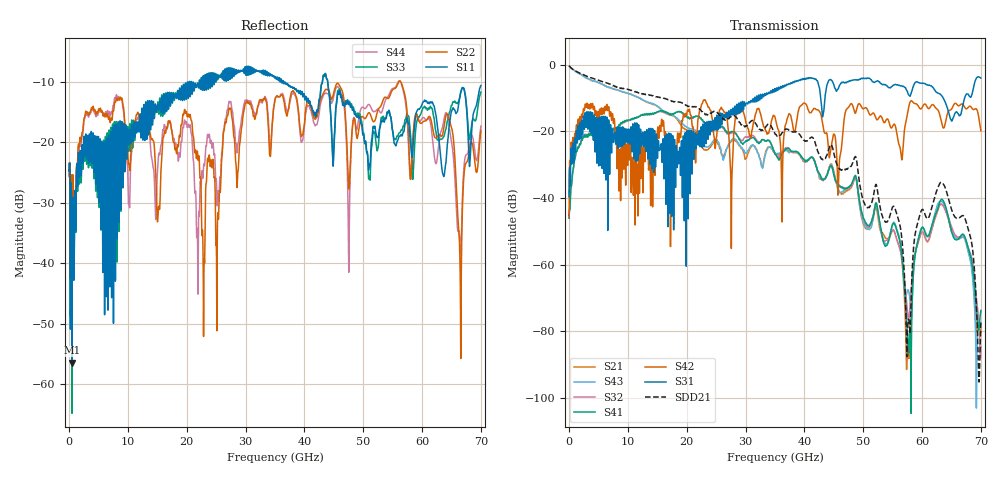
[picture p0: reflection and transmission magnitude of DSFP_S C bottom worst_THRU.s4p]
! AWR Design Environment (8415) Wed Jan 09 13:26:57 2019
! Document = 'DSFP_S'
! nPorts: 4, nXvals: 7001
# HZ S DB R 50
!Freq DBS11 AngS11 DBS12 AngS12 DBS13 AngS13 DBS14 AngS14
!	DBS21 AngS21 DBS22 AngS22 DBS23 AngS23 DBS24 AngS24
!	DBS31 AngS31 DBS32 AngS32 DBS33 AngS33 DBS34 AngS34
!	DBS41 AngS41 DBS42 AngS42 DBS43 AngS43 DBS44 AngS44
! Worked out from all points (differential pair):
!   7000 points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, 10 MHz to 70 GHz, reference 50 ohm
!   strongest paths, dB at 10 MHz, 17.51 GHz, 35.01 GHz, 52.51 GHz, 70 GHz:
!     S31: -39.6, -26.7, -7.3, -4.9, -4.0
!     S42: -45.6, -25.7, -15.8, -16.4, -19.9
!     S41: -46.1, -14.9, -26.7, -44.1, -73.8
!     S32: -45.2, -15.0, -26.7, -45.2, -84.7
!     S43: -0.5, -15.1, -26.7, -44.5, -77.4
!     S21: -0.5, -15.3, -26.9, -46.0, -79.6
!   taken as a pair (ports 3,1 in; 4,2 out), SDD21 dB: -0.4, -11.1, -20.8, -38.9, -77.0
!   lowest |S11| = -56.5 dB at 500 MHz (marker M1), VSWR 1.00, Z = 50 + j0.146 ohm
!   |S11| at or under -10 dB: start of sweep to 20.42 GHz; 36.43 GHz to 43.08 GHz (6.652 GHz wide, 16.7 % of centre); 43.95 GHz to end of sweep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
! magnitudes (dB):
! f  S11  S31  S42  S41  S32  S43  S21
! 10 MHz  -24.7  -39.6  -45.6  -46.1  -45.2  -0.5  -0.5
! 500 MHz  -56.5  -29.8  -25.4  -34.2  -34.4  -1.3  -1.3
! 33.87 GHz  -8.6  -8.5  -20.7  -22.8  -22.8  -24.9  -24.7
! 55.35 GHz  -20.3  -6.0  -18.0  -47.9  -50.3  -47.5  -50.4
! 57.82 GHz  -17.5  -9.3  -12.0  -81.6  -75.2  -68.8  -87.1
! 63.51 GHz  -25.2  -9.8  -18.7  -40.6  -42.2  -41.3  -42.1
! 70 GHz  -10.7  -4.0  -19.9  -73.8  -84.7  -77.4  -79.6
